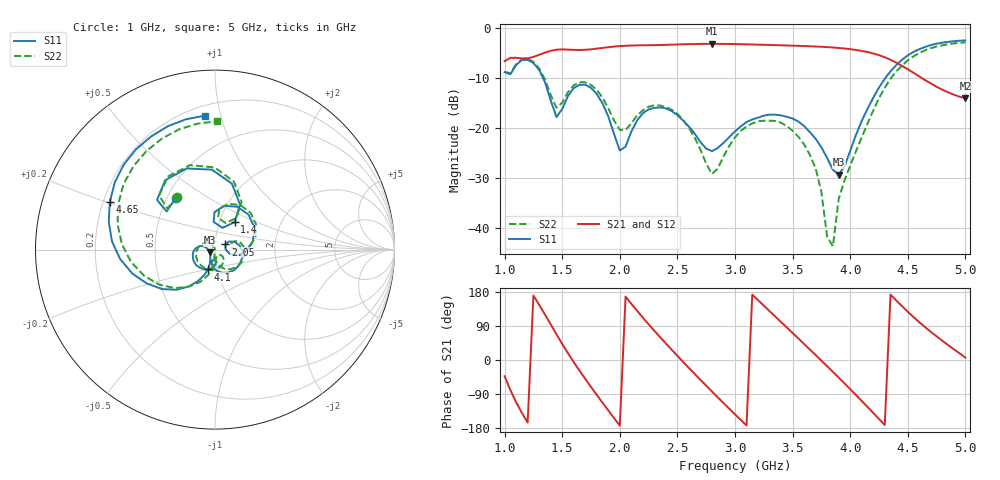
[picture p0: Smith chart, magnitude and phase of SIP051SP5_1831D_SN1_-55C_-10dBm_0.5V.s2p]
# GHz  S  dB  R  50
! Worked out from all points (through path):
!   81 points, 1 GHz to 5 GHz, reference 50 ohm
!   highest |S21| = -3.19 dB at 2.8 GHz (marker M1); lowest = -14.1 dB at 5 GHz (marker M2)
!   lowest |S11| = -29.3 dB at 3.9 GHz (marker M3), VSWR 1.07, Z = 47 - j1.42 ohm
!   |S11| at or under -10 dB: 1.333 GHz to 4.306 GHz (2.973 GHz wide, 105 % of centre)
!   |S22| runs from -43.7 to -2.9 dB; largest |S21 - S12| = 0.0024
!   S11 on the Smith chart (normalised r, x): 1 GHz: 0.55, +0.37; 1.4 GHz: 1.18, +0.38; 2.05 GHz: 1.12, +0.06; 4.1 GHz: 0.90, -0.20; 4.65 GHz: 0.23, +0.21; 5 GHz: 0.26, +0.89
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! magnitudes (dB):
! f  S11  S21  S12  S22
! 1 GHz  -8.8  -6.7  -6.6  -8.8
! 1.25 GHz  -7.0  -5.8  -5.8  -6.8
! 1.4 GHz  -14.5  -4.6  -4.6  -13.4
! 1.45 GHz  -17.8  -4.4  -4.4  -16.0
! 1.7 GHz  -11.4  -4.4  -4.4  -10.9
! 1.85 GHz  -15.1  -4.0  -4.0  -14.0
! 2 GHz  -24.6  -3.6  -3.6  -20.4
! 2.05 GHz  -23.8  -3.6  -3.6  -20.4
! 2.2 GHz  -17.1  -3.5  -3.5  -16.5
! 2.35 GHz  -15.9  -3.4  -3.4  -15.5
! 2.55 GHz  -18.6  -3.3  -3.3  -18.4
! 2.8 GHz  -24.7  -3.2  -3.2  -29.2
! 3 GHz  -20.7  -3.2  -3.2  -21.9
! 3.4 GHz  -17.5  -3.5  -3.5  -19.0
! 3.7 GHz  -22.2  -3.7  -3.7  -28.1
! 3.8 GHz  -26.0  -3.9  -3.9  -41.8
! 3.85 GHz  -28.4  -3.9  -3.9  -43.7
! 3.9 GHz  -29.3  -4.0  -4.0  -34.2
! 4.1 GHz  -18.6  -4.6  -4.6  -21.9
! 4.35 GHz  -8.7  -6.4  -6.4  -10.2
! 4.65 GHz  -3.8  -10.4  -10.4  -4.5
! 5 GHz  -2.5  -14.1  -14.1  -2.9
